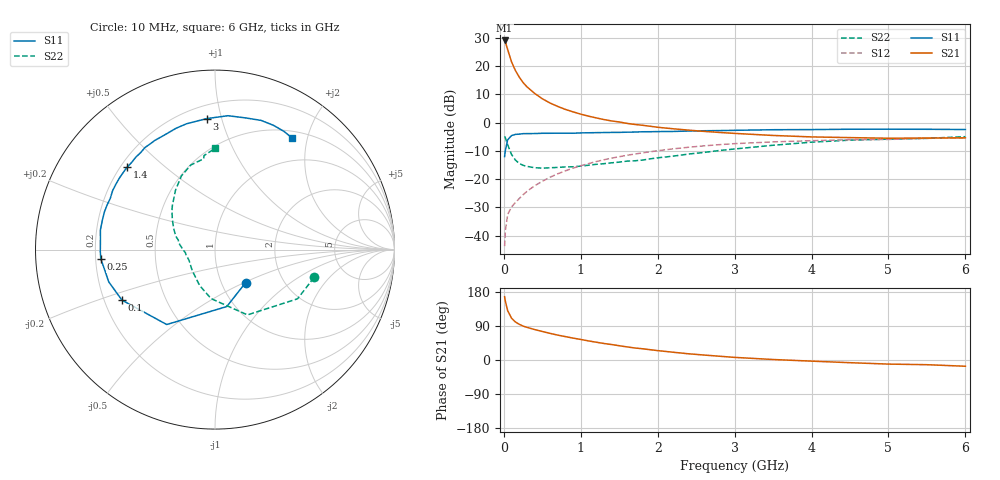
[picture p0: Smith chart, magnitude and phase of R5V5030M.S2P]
! SIEMENS Small Signal Semiconductors
! BFR183
! Si NPN RF Bipolar Junction Transistor in SOT23
! VCE = 0.5 V  IC = 30 mA
! Common Emitter S-Parameters:  May  1996
# GHz  S  MA  R  50
!  f  S11  S21  S12  S22
! GHz  MAG  ANG  MAG  ANG  MAG  ANG  MAG  ANG
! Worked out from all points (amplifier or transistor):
!   36 points, 10 MHz to 6 GHz, reference 50 ohm
!   highest |S21| = 29.1 dB at 10 MHz (marker M1)
!   |S21| within 3 dB of that: start of sweep to 47.22 MHz
!   unconditionally stable (mu >= 1): start of sweep to 19.61 MHz; 140.5 MHz to end of sweep
!   at 250 MHz: K = 1.21, MAG = 17.1 dB, |S12| = -25.5 dB
!   at 1.4 GHz: K = 1.28, MAG = 3.4 dB, |S12| = -12.6 dB
!   at 6 GHz: K = 1.08, MAG = -1.7 dB, |S12| = -5.4 dB
!   S11 on the Smith chart (normalised r, x): 10 MHz: 1.30, -0.51; 100 MHz: 0.27, -0.24; 250 MHz: 0.22, -0.04; 1.4 GHz: 0.23, +0.38; 3 GHz: 0.29, +0.90; 6 GHz: 0.60, +1.75
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0.01  0.2511 -47.2  28.52 166.9  0.0065 70.1  0.5736 -15.7
0.02  0.324 -78.3  26.78 155.0  0.0123 66.8  0.5354 -30.8
0.05  0.4966 -122.8  19.61 130.1  0.0237 55.1  0.4062 -63.6
0.1  0.5899 -151.5  11.93 110.3  0.0321 51.7  0.2739 -94.6
0.15  0.6188 -163.1  8.388 100.4  0.0385 53.9  0.2177 -113.2
0.2  0.6261 -170.2  6.414 94.3  0.0453 57.6  0.1893 -124.6
0.25  0.6384 -175.4  5.127 89.5  0.0528 59.8  0.1757 -134.4
0.3  0.6391 -179.0  4.318 86.2  0.0606 62.1  0.1679 -141.1
0.4  0.641 174.7  3.297 80.4  0.0762 64.0  0.1594 -150.3
0.5  0.6479 170.2  2.649 75.3  0.0916 65.1  0.1565 -157.5
0.6  0.6486 165.2  2.226 70.3  0.108 65.0  0.1587 -162.7
0.7  0.6508 161.3  1.937 65.7  0.1241 64.6  0.1613 -166.7
0.9  0.6493 154.0  1.552 57.8  0.1566 62.7  0.1654 -173.5
1.1  0.6613 146.8  1.303 50.4  0.1882 60.1  0.1763 -178.6
1.4  0.6712 136.7  1.072 40.8  0.235 55.3  0.1943 173.4
1.7  0.6811 127.3  0.93 31.8  0.2775 50.3  0.2109 165.5
2.2  0.6982 113.4  0.779 20.5  0.3436 41.4  0.2551 153.8
3  0.7312 93.7  0.645 6.9  0.4246 26.8  0.3419 134.0
3.5  0.7494 84.5  0.593 1.3  0.4564 18.5  0.3975 123.6
4.5  0.7643 70.3  0.543 -7.1  0.4979 4.5  0.4899 106.1
5.5  0.7626 59.8  0.534 -12.4  0.527 -5.7  0.5271 96.7
6  0.7556 55.3  0.538 -16.5  0.5362 -12.3  0.5647 89.9
